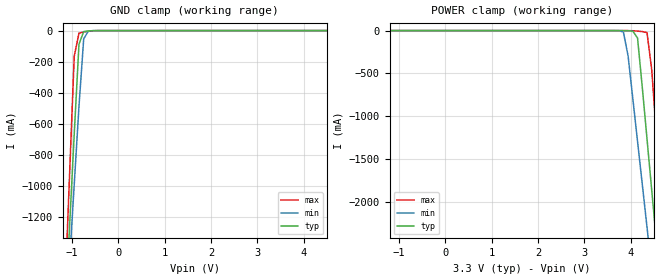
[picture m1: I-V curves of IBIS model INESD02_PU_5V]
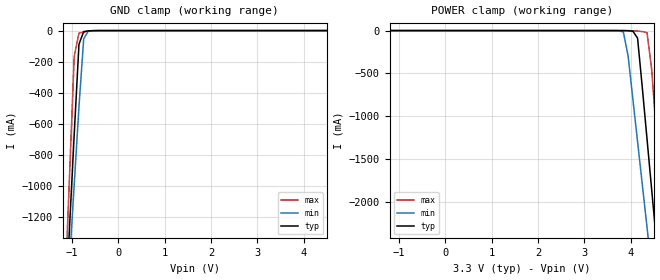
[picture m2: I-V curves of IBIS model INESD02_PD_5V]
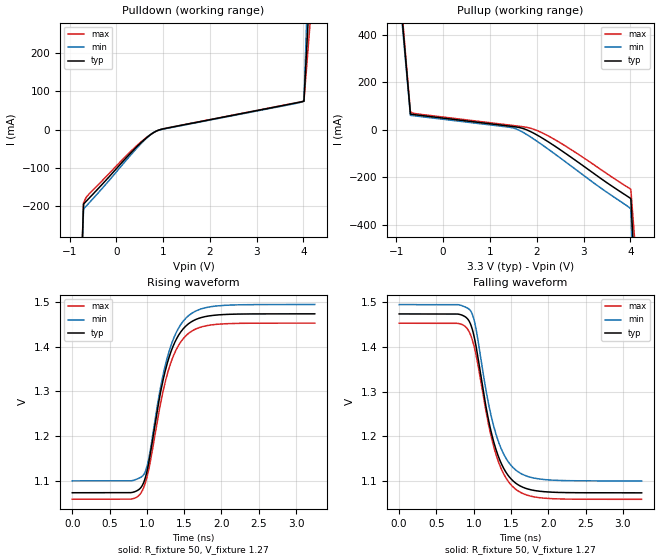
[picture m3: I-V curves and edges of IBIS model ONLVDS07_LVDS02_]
|   This file is an IBIS representation of the   |
|   Integrated Device Technology, Inc   |
|   ICS854105   |
|   LOW SKEW, 1-TO-4, LVCMOS/LVTTL-TO-LVDS FANOUT BUFFER   |
[IBIS Ver]   4.1
[File name]   854105_3v3.ibs
[File Rev]   1.0
[Date]   13 May 2010
[Source]   Originated at Integrated Device Technology, Inc.
[Disclaimer]
IDT hereby grants the user of this IBIS model a non-exclusive,
nontransferable license to use this IBIS model under the following terms.
Before using this IBIS model, the user should read this license.
If the user does not accept these terms,  the IBIS model should be
returned to IDT within 30 days.
   The user is granted this license only to use the IBIS model and
is not granted rights to sell, load, rent, lease or license the IBIS
model in whole or in part, or in modified form to anyone other than
user. User may modify the IBIS model to suit its specific
applications but rights to derivative works and such modifications
shall belong to IDT.
   This IBIS model is provided on an "AS IS" basis and IDT makes
absolutely no warranty with respect to the information contained
herein. IDT DISCLAIMS AND CUSTOMER WAIVES ALL WARRANTIES, EXPRESS
OR IMPLIED, INCLUDING WARRANTIES OF MERCHANTABILITY OR FITNESS FOR
A PARTICULAR PURPOSE. The entire risk as to quality and performance
is with the Customer. ACCORDINGLY, IN NO EVENT SHALL THE COMPANY BE
LIABLE FOR ANY DAMAGES, WHETHER IN CONTRACT OR TORT,INCLUDING ANY
LOST PROFITS OR OTHER INCIDENTAL, CONSEQUENTIAL, EXEMPLARY, OR
PUNITIVE DAMAGES ARISING OUT OF THE USE OR APPLICATION OF THE IBIS
model provided in this package. Further, IDT reserves the right to
make changes without notice to any product herein to improve
reliability, function, or design. IDT does not convey any license
under patent rights or any other intellectual property rights,
including those of third parties.
   IDT is not obligated to provide maintenance or support
for the licensed IBIS model.
[Copyright]   Copyright 2010 by Integrated Device Technology, Inc.
[Component]   ICS854105G
[Manufacturer] Integrated Device Technology, Inc.
[Package]
|   TSSOP16   typ   min   max
R_pkg   58.65m   52.5m   64.8m
L_pkg   1.902nH   1.443nH   2.361nH
C_pkg   0.315pF   0.254pF   0.375pF
[Pin] signal_name   model_name   R_pin   L_pin   C_pin
1  OE0   INESD02_PU_5V   64.8m   2.361n   0.375p
2  OE1   INESD02_PU_5V   60.7m   2.054n   0.335p
3  OE2   INESD02_PU_5V   56.6m   1.749n   0.294p
4  VDD   POWER   52.5m   1.443n   0.254p
5  GND   GND   52.5m   1.443n   0.254p
6  CLK   INESD02_PD_5V   56.6m   1.749n   0.294p
7  NC   NC   60.7m   2.054n   0.335p
8  OE3   INESD02_PU_5V   64.8m   2.361n   0.375p
9  nQ3   ONLVDS07_LVDS02_   64.8m   2.361n   0.375p
10 Q3   ONLVDS07_LVDS02_   60.7m   2.054n   0.335p
11 nQ2   ONLVDS07_LVDS02_   56.6m   1.749n   0.294p
12 Q2   ONLVDS07_LVDS02_   52.5m   1.443n   0.254p
13 nQ1   ONLVDS07_LVDS02_   52.5m   1.443n   0.254p
14 Q1   ONLVDS07_LVDS02_   56.6m   1.749n   0.294p
15 nQ0   ONLVDS07_LVDS02_   60.7m   2.054n   0.335p
16 Q0   ONLVDS07_LVDS02_   64.8m   2.361n   0.375p
[Diff Pin]  inv_pin  vdiff tdelay_typ tdelay_min  tdelay_max
10   9   NA   0   0   0
12   11   NA   0   0   0
14   13   NA   0   0   0
16   15   NA   0   0   0
| Models and submodels in the file (3): INESD02_PU_5V (Input), INESD02_PD_5V (Input), ONLVDS07_LVDS02_ (Output)
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[Model]   INESD02_PU_5V
Model_type   Input
Polarity   Non-Inverting
Vinl = 0.8V
Vinh = 2.0V
|   typ   min   max
C_comp   2pF   1.5pF   2.5pF
|   typ   min   max
[Voltage range]  3.3V   3.135V   3.465V
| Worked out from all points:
|   GND clamp passes 1 mA (typ) near -0.58 V on its own axis
[GND_clamp]
|Voltage   I(typ)   I(min)   I(max)
-3.3V     -14.52A    -12.53A    -17.87A
-1.157V   -1.867A    -1.989A    -1.704A
-1.055V   -1.265A    -1.488A    -934.1mA
-952.6mV  -663.5mA   -987.5mA   -164.6mA
-850.5mV  -87.67mA   -487.6mA   -16.09mA
-748.5mV  -6.381mA   -52.8mA    -9.221mA
-646.4mV  -1.974mA   -2.739mA   -4.198mA
-340.2mV  -74.07uA   -86.47uA   -63.25uA
6.6V      64.29uA    84.42uA    47.33uA
[POWER_clamp]
|Voltage   I(typ)   I(min)   I(max)
-3.3V     64.29uA    80.4uA     49.82uA
3.64V     -74.07uA   -182uA     -54.96uA
3.844V    -481.8uA   -15.93mA   -77.98uA
3.946V    -1.974mA   -296.1mA   -341uA
4.048V    -6.381mA   -795.8mA   -1.985mA
4.151V    -87.67mA   -1.296A    -5.959mA
4.355V    -1.265A    -2.297A    -23.88mA
4.457V    -1.867A    -2.799A    -459.4mA
4.559V    -2.47A     -3.3A      -1.229A
4.661V    -3.072A    -3.801A    -1.999A
4.763V    -3.675A    -4.303A    -2.769A
6.6V      -14.52A    -13.34A    -16.63A
[Model]   INESD02_PD_5V
Model_type  Input
Polarity   Non-Inverting
Vinl = 0.8V
Vinh = 2.0V
|   typ   min   max
C_comp   2pF   1.5pF   2.5pF
|   typ   min   max
[Voltage range]  3.3V   3.135V   3.465V
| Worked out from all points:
|   GND clamp passes 1 mA (typ) near -0.58 V on its own axis
[GND_clamp]
|Voltage   I(typ)   I(min)   I(max)
-1.973V   -6.688A    -6A        -7.863A
-1.157V   -1.867A    -1.988A    -1.704A
-1.055V   -1.265A    -1.488A    -934.1mA
-952.6mV  -663.4mA   -987.4mA   -164.5mA
-850.5mV  -87.6mA    -487.5mA   -16.04mA
-748.5mV  -6.317mA   -52.72mA   -9.171mA
-646.4mV  -1.91mA    -2.66mA    -4.148mA
-340.2mV  -9.776uA   -8.593uA   -12.08uA
6.6V      128.6uA    131.6uA    121.8uA
[POWER_clamp]
|Voltage   I(typ)   I(min)   I(max)
-3.3V     128.6uA    128.3uA    124.8uA
3.64V     -9.776uA   -103.4uA   -3.241uA
3.844V    -417.5uA   -15.85mA   -26.94uA
3.946V    -1.91mA    -296.1mA   -290.3uA
4.048V    -6.317mA   -795.7mA   -1.934mA
4.151V    -87.6mA    -1.296A    -5.908mA
4.355V    -1.265A    -2.297A    -23.83mA
4.457V    -1.867A    -2.799A    -459.4mA
4.559V    -2.47A     -3.3A      -1.229A
4.661V    -3.072A    -3.801A    -1.999A
4.763V    -3.675A    -4.303A    -2.769A
5.681V    -9.099A    -8.82A     -9.698A
[Model]   ONLVDS07_LVDS02_
Model_type   Output
Polarity   Non-Inverting
|   typ   min   max
C_comp   2pF   1.5pF   2.5pF
Vmeas = 1.27V
Rref = 50
Cref = 0
Vref = 1.27V
|   typ   min   max
[Voltage range]   3.3V   3.135V   3.465V
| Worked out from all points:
|   slope of the pulldown table from 0 to 0.495 V, typ, clamps not added: 7.72 ohm
|   slope of the pullup table from 0 to 0.495 V, typ, clamps not added: 42.1 ohm
|   rising waveform, R_fixture 50, V_fixture 1.27: 20-80 % time 294ps typ, 295ps min, 303ps max; typ from 1.07 V to 1.47 V
|   falling waveform, R_fixture 50, V_fixture 1.27: 20-80 % time 294ps typ, 295ps min, 303ps max; typ from 1.47 V to 1.07 V
[Pulldown]
|Voltage   I (typ)   I (min)   I (max)
-3.3V     -12.65A    -15.46A    -10.98A
-1.22V    -2.111A    -2.068A    -2.153A
-700mV    -193.8mA   -206.5mA   -190.5mA
-645mV    -186.6mA   -199.2mA   -176.4mA
-591mV    -179.6mA   -192mA     -168.6mA
381.2mV   -51.39mA   -55.77mA   -47.77mA
651.3mV   -20.4mA    -21.4mA    -19.48mA
813.3mV   -6.203mA   -5.872mA   -6.355mA
1.083V    4.273mA    3.578mA    4.591mA
4.01V     74.38mA    74.89mA    74.44mA
4.528V    1.282A     1.92A      877.3mA
6.6V      7.966A     10.44A     6.456A
[Pullup]
|Voltage   I (typ)   I (min)   I (max)
-3.3V     7.958A     9.751A     6.893A
-1.22V    1.248A     1.203A     1.29A
-700mV    66.02mA    60.62mA    74.84mA
-537mV    61.66mA    56.73mA    66.33mA
1.461V    14.18mA    8.952mA    18.64mA
1.623V    9.51mA     -2.335mA   14.76mA
1.786V    -533.3uA   -20.17mA   10.05mA
2.164V    -40.74mA   -70.36mA   -17.8mA
2.704V    -111.8mA   -148.4mA   -79.91mA
4.01V     -290.1mA   -334mA     -250.7mA
4.528V    -2.246A    -3.273A    -1.583A
6.6V      -12.68A    -16.56A    -10.3A
[Ramp]
|   typ   min   max
dV/dt_r   0.321/0.466n   0.316/0.465n   0.316/0.481n
dV/dt_f   0.321/0.466n   0.316/0.465n   0.316/0.481n
R_load =   50.0000
[Rising Waveform]
R_fixture = 50
V_fixture = 1.27   |Vcc_typ
V_fixture_min = 1.285 |Vcc_min
V_fixture_max = 1.26  |Vcc_max
C_fixture = 0.0p
| Time   typ   min   max
0s        1.073V     1.099V     1.058V
793.8ps   1.073V     1.1V       1.059V
956.5ps   1.095V     1.113V     1.084V
1.025ns   1.14V      1.149V     1.125V
1.171ns   1.288V     1.298V     1.262V
1.275ns   1.364V     1.377V     1.34V
1.405ns   1.42V      1.436V     1.397V
1.565ns   1.453V     1.471V     1.431V
1.965ns   1.472V     1.492V     1.451V
3.25ns    1.474V     1.495V     1.453V
[Falling Waveform]
R_fixture = 50
V_fixture = 1.27   |Vcc_typ
V_fixture_min = 1.285 |Vcc_min
V_fixture_max = 1.26  |Vcc_max
C_fixture = 0.0p
| Time   typ   min   max
0s        1.474V     1.495V     1.453V
793.8ps   1.474V     1.495V     1.453V
956.5ps   1.451V     1.481V     1.427V
1.025ns   1.407V     1.445V     1.387V
1.171ns   1.259V     1.296V     1.249V
1.275ns   1.183V     1.217V     1.172V
1.405ns   1.126V     1.158V     1.114V
1.565ns   1.094V     1.124V     1.08V
1.965ns   1.075V     1.102V     1.061V
3.25ns    1.073V     1.099V     1.058V
